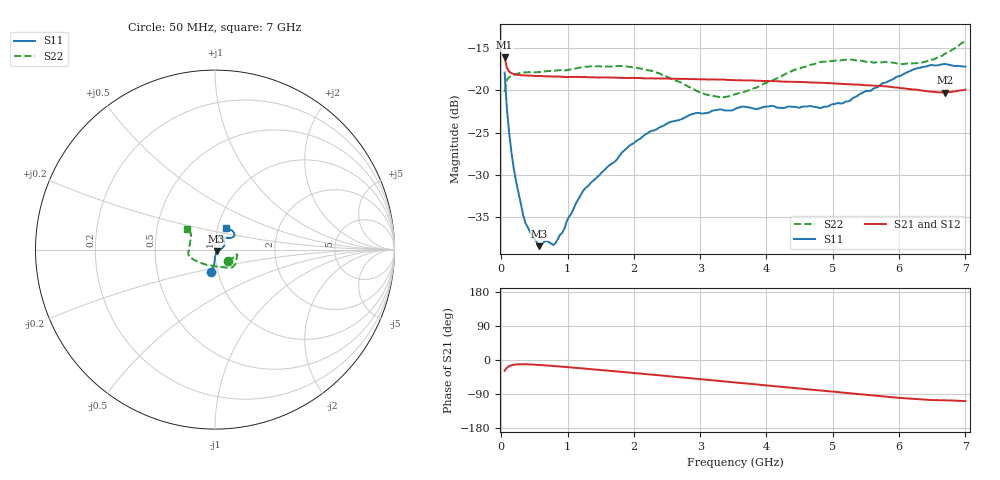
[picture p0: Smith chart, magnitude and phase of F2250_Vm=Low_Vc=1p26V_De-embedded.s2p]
! Integrated Device Technology
! Corporate Headquarters
! 6024 Silver Creek Valley Road
! San Jose, CA 95138  USA
! Phone:  1-408-284-8200
! Toll Free:  1-800-223-1366
! Webpage:  http://www.idt.com/
! Timing and RF Division
! 515 Groton Road, Suite 102
! Westford, MA 01886-6024
! Device:  F2250
! Description: Voltage Variable RF Attenuator
! Frequency:  50.0 -  6000.00 MHz
! Package:  3x3 mm Thin QFN Plastic Package: 16 pin
! Ports:  2 RF, 3 DC
!  Pin  1  = GND
!  Pin  2  = NC
!  Pin  3  = RF1  = Port 1
!  Pin  4  = NC
!  Pin  5  = GND
!  Pin  6  = GND
!  Pin  7  = GND
!  Pin  8  = GND
!  Pin  9  = NC
!  Pin 10  = RF2  = Port 2
!  Pin 11  = NC
!  Pin 12  = GND
!  Pin 13  = GND
!  Pin 14  = VCNTRL
!  Pin 15  = VDD
!  Pin 16  = VMODE
! Vcntrl:  1.260 Volts
! Vmode:  +0.000 Volts
! Vdd:  +3.30  Volts
! Current:  1.193 mA
! Data:  The device was measured on a the F2250 evaluation board which has
!  individual transmission lines to the RF pins.  Data was collected
!  using a calibrated network analyzer.  The evaluation board was
!  de-embedded using a TRL calibration technique.
!  The reference plane is the edge of the package pin.
! Misc:  SN 10
!  Action Tracker AT0258
! Date Measured:  2014-11-26
! Date:  2015-10-15  MJV
! Note:
!  Integrated Device Technology supplies this data as a sample of measured
!  data at the package pin for this product.  Your particular data for this
!  product may vary.
!  Data was taken at 25 degrees C.
!  Integrated Device Technology reserves the right to change this data at anytime.
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# GHz S dB R 50
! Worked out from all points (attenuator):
!   201 points, 50 MHz to 7 GHz, reference 50 ohm
!   highest |S21| = -16.12 dB at 50 MHz (marker M1); lowest = -20.3 dB at 6.687 GHz (marker M2)
!   lowest |S11| = -38.4 dB at 571.2 MHz (marker M3), VSWR 1.02, Z = 50.9 - j0.812 ohm
!   |S11| at or under -10 dB: start of sweep to end of sweep
!   |S22| runs from -20.8 to -14.1 dB; largest |S21 - S12| = 0.00043
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0.05  -17.90 -99.1  -16.12 -28.3  -16.10 -28.3  -20.19 -41.5
0.08475  -22.19 -92.4  -17.36 -20.2  -17.37 -20.2  -18.75 -20.2
0.1195  -25.12 -91.1  -17.81 -16.1  -17.80 -16.1  -18.47 -14.5
0.15425  -27.40 -90.2  -17.98 -13.8  -17.97 -13.8  -18.35 -12.8
0.22375  -30.83 -82.8  -18.16 -11.8  -18.16 -11.8  -18.11 -12.4
0.36275  -35.66 -70.8  -18.26 -11.3  -18.25 -11.3  -17.90 -13.1
0.57125  -38.43 -41.7  -18.32 -13.0  -18.32 -13.0  -17.86 -18.0
0.6755  -37.81 -35.8  -18.35 -14.3  -18.36 -14.3  -17.75 -20.6
0.8145  -38.13 -21.0  -18.39 -16.2  -18.38 -16.2  -17.69 -24.5
1.2315  -31.93 -5.1  -18.45 -22.3  -18.42 -22.3  -17.26 -34.1
1.9265  -26.58 16.4  -18.55 -33.1  -18.56 -33.1  -17.23 -45.3
2.37825  -24.43 27.7  -18.61 -40.3  -18.61 -40.4  -17.99 -53.8
2.86475  -22.85 42.7  -18.68 -48.3  -18.68 -48.3  -19.74 -70.4
3.07325  -22.72 49.4  -18.71 -51.8  -18.72 -51.7  -20.48 -81.7
3.3165  -22.26 57.7  -18.74 -55.8  -18.75 -55.8  -20.83 -98.2
3.525  -22.23 62.4  -18.82 -59.2  -18.83 -59.2  -20.48 -112.5
4.7065  -21.97 67.5  -19.09 -78.9  -19.08 -78.9  -16.94 -161.3
5.22775  -21.33 50.5  -19.28 -87.5  -19.27 -87.6  -16.41 -170.9
5.85325  -18.88 35.4  -19.59 -97.7  -19.60 -97.7  -16.74 175.6
6.33975  -17.29 37.6  -20.04 -104.3  -20.05 -104.4  -16.72 158.4
6.68725  -16.90 46.6  -20.28 -106.4  -20.26 -106.5  -15.70 145.9
7  -17.20 62.9  -19.93 -108.5  -19.94 -108.6  -14.12 143.3
